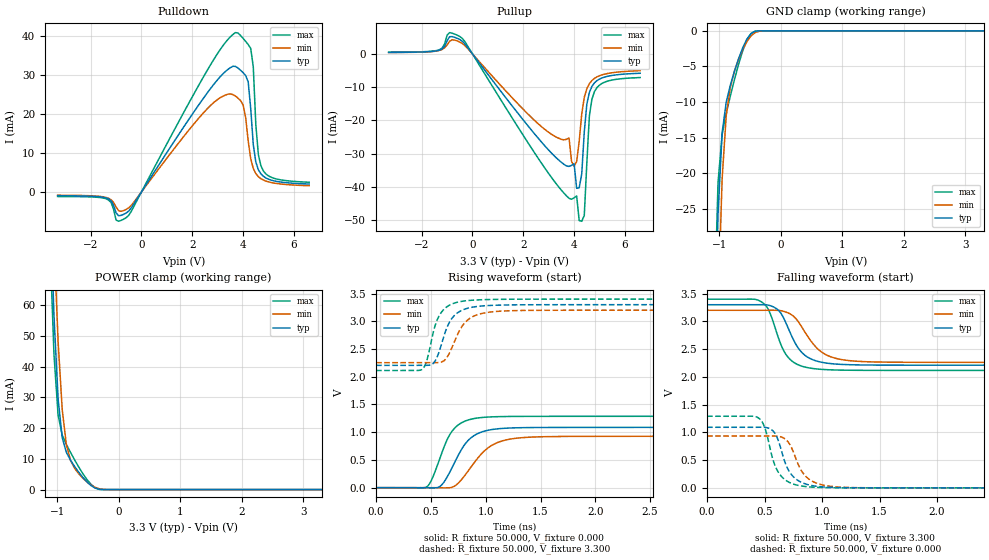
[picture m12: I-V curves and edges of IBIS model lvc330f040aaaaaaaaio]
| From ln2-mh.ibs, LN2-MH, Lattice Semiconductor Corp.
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|   Model lvc330f040aaaaaaaaio
[Model] lvc330f040aaaaaaaaio
Model_type I/O
Polarity   Non-Inverting
Enable   Active-Low
Vinl =  0.800V
Vinh =  2.000V
Vmeas =  1.650V
Cref =  0.0F
Rref =  1.000M
Vref =  0.0V
C_comp   2.000pF   1.500pF   2.500pF
[Temperature Range]   25.000   0.125k   -40.000
[Voltage Range]   3.300V   3.200V   3.400V
[C Comp Corner]
C_comp   2.000pF   1.500pF   2.500pF
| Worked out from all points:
|   slope of the pulldown table from 0 to 0.495 V, typ, clamps not added: 98.5 ohm
|   slope of the pullup table from 0 to 0.495 V, typ, clamps not added: 98.9 ohm
|   GND clamp passes 1 mA (typ) near -0.54 V on its own axis
|   POWER clamp passes 1 mA (typ) near -0.43 V on its own axis
|   rising waveform, R_fixture 50.000, V_fixture 0.000: 20-80 % time 196ps typ, 247ps min, 167ps max; typ from 0 V to 1.09 V
|   rising waveform, R_fixture 50.000, V_fixture 3.300: 20-80 % time 133ps typ, 155ps min, 115ps max; typ from 2.21 V to 3.3 V
|   falling waveform, R_fixture 50.000, V_fixture 3.300: 20-80 % time 171ps typ, 212ps min, 149ps max; typ from 3.3 V to 2.21 V
|   falling waveform, R_fixture 50.000, V_fixture 0.000: 20-80 % time 127ps typ, 140ps min, 117ps max; typ from 1.09 V to 0 V
[Pulldown]
|Voltage   I(typ)   I(min)   I(max)
-3.3V     -991.1uA   -858.3uA   -1.183mA
-600mV    -5.406mA   -4.489mA   -6.6mA
2.6V      25.49mA    21.41mA    31.32mA
3.7V      32.19mA    24.56mA    40.89mA
4V        30.59mA    22.3mA     39.39mA
4.2V      28.23mA    13.08mA    37.81mA
4.3V      21.31mA    8.471mA    36.8mA
4.4V      12.1mA     6.034mA    32.08mA
4.5V      7.681mA    4.709mA    17.27mA
4.6V      5.686mA    3.907mA    9.552mA
4.8V      3.997mA    3.033mA    5.35mA
6.6V      2.008mA    1.58mA     2.473mA
[Pullup]
|Voltage   I(typ)   I(min)   I(max)
-3.3V     467.7uA    422.2uA    537.6uA
-400mV    3.822mA    3.145mA    4.669mA
2.6V      -25.45mA   -21.08mA   -31.53mA
3.8V      -33.81mA   -25.27mA   -43.4mA
4V        -33mA      -33.77mA   -43.26mA
4.1V      -40.39mA   -32.36mA   -42.69mA
4.3V      -36.05mA   -18.05mA   -50.31mA
4.4V      -23.44mA   -13.06mA   -48.55mA
4.5V      -15.1mA    -10.46mA   -32.86mA
4.6V      -11.58mA   -8.931mA   -18.68mA
4.8V      -8.69mA    -7.351mA   -11.32mA
6.6V      -5.804mA   -5.021mA   -7.09mA
[GND_clamp]
|Voltage   I(typ)   I(min)   I(max)
-3.3V     -1.861A    -1.855A    -1.868A
-1.089V   -50.81mA   -68.2mA    -41.77mA
-1.022V   -25.74mA   -39.08mA   -21.31mA
-955mV    -14.26mA   -20.73mA   -14.54mA
-888mV    -9.982mA   -11.84mA   -11.55mA
-821mV    -7.603mA   -7.856mA   -9.113mA
-754mV    -5.655mA   -5.623mA   -6.821mA
-620mV    -2.371mA   -2.616mA   -2.797mA
-553mV    -1.172mA   -1.518mA   -1.313mA
-486mV    -396.2uA   -716.4uA   -376.4uA
-419mV    -71.95uA   -244.9uA   -42.84uA
3.3V      0A         0A         0A
[POWER_clamp]
|Voltage   I(typ)   I(min)   I(max)
-3.266V   2.002A     2.005A     2.003A
-1.122V   95.84mA    122.3mA    80.75mA
-1.055V   56.42mA    81.13mA    43.84mA
-988mV    29.46mA    48.05mA    24.15mA
-921mV    16.84mA    25.99mA    17.71mA
-854mV    12.12mA    14.6mA     14.67mA
-787mV    9.585mA    9.535mA    12.12mA
-720mV    7.529mA    6.931mA    9.676mA
-519mV    2.487mA    2.496mA    3.276mA
-385mV    477.3uA    731.6uA    579.8uA
-184mV    1.009uA    11.15uA    276.7nA
3.3V      0A         0A         0A
[Ramp]
| variable   typ   min   max
dV/dt_r   0.669/0.196n   0.572/0.247n   0.790/0.168n
dV/dt_f   0.670/0.172n   0.580/0.213n   0.788/0.150n
R_load = 50.000
[Rising Waveform]
R_fixture = 50.000
V_fixture = 0.000
V_fixture_min = 0.000
V_fixture_max = 0.000
|  time   V(typ)   V(min)   V(max)
0s        3.936uV    16.32uV    1.484uV
457ps     -1.109mV   -256.1uV   9.158mV
507ps     -3.239mV   -147uV     143.1mV
571ps     9.294mV    -1.823mV   467.4mV
665ps     252.8mV    -1.792mV   930.1mV
761ps     626mV      104.4mV    1.147V
922ps     970mV      518.6mV    1.255V
1.051ns   1.046V     757.4mV    1.276V
1.202ns   1.074V     867.8mV    1.284V
50ns      1.092V     934.2mV    1.29V
[Rising Waveform]
R_fixture = 50.000
V_fixture = 3.300
V_fixture_min = 3.200
V_fixture_max = 3.400
|  time   V(typ)   V(min)   V(max)
0s        2.206V     2.254V     2.113V
428ps     2.207V     2.255V     2.147V
467ps     2.207V     2.255V     2.322V
531ps     2.262V     2.255V     2.87V
601ps     2.615V     2.269V     3.176V
667ps     2.975V     2.42V      3.288V
750ps     3.162V     2.788V     3.348V
868ps     3.251V     3.069V     3.379V
1.097ns   3.291V     3.178V     3.395V
50ns      3.3V       3.2V       3.4V
[Falling Waveform]
R_fixture = 50.000
V_fixture = 3.300
V_fixture_min = 3.200
V_fixture_max = 3.400
|  time   V(typ)   V(min)   V(max)
0s        3.3V       3.2V       3.4V
479ps     3.301V     3.2V       3.342V
539ps     3.289V     3.2V       3.188V
610ps     3.219V     3.199V     2.768V
683ps     2.984V     3.17V      2.413V
777ps     2.57V      3.038V     2.233V
858ps     2.378V     2.784V     2.174V
1.003ns   2.26V      2.438V     2.134V
1.203ns   2.222V     2.301V     2.12V
50ns      2.206V     2.254V     2.113V
[Falling Waveform]
R_fixture = 50.000
V_fixture = 0.000
V_fixture_min = 0.000
V_fixture_max = 0.000
|  time   V(typ)   V(min)   V(max)
0s        1.092V     934.2mV    1.29V
458ps     1.093V     933.9mV    1.242V
509ps     1.088V     934mV      1.04V
578ps     1.016V     934.3mV    475.5mV
651ps     638.6mV    912.6mV    197.2mV
703ps     338.5mV    831.6mV    112.2mV
780ps     148.1mV    485.3mV    50.67mV
887ps     52.22mV    156.1mV    17.68mV
1.087ns   8.284mV    25.14mV    2.75mV
50ns      3.936uV    16.32uV    1.484uV
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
